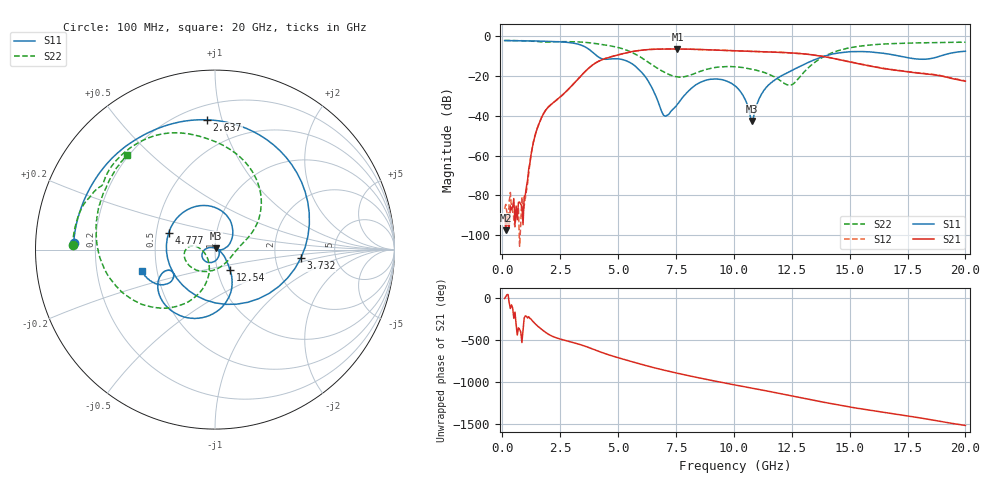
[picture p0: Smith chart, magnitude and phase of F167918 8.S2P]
!  2-Port S-parameters saved by WinCal
! VAR MeasName=S-Parameters (CALIBRATED_DATA) read from VNA (N5242A)
! VAR MeasDate=2016-11-22 10:25:13
! VAR NAME=F167918 8
! VAR FILENAME=F167918 8.S2P
! VAR DATE=2016-11-22 10:25:13
! VAR PHYS_PORTS=1,2
# Hz S DB R 50
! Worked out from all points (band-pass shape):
!   401 points, 100 MHz to 20 GHz, reference 50 ohm
!   highest |S21| = -6.30 dB at 7.562 GHz (marker M1); lowest = -97.6 dB at 149.8 MHz (marker M2)
!   |S21| within 3 dB of the highest: 4.991 GHz to 13.42 GHz (8.428 GHz wide, 91.6 % of centre)
!   lowest |S11| = -42.5 dB at 10.8 GHz (marker M3), VSWR 1.02, Z = 50.4 + j0.636 ohm
!   |S11| at or under -10 dB: 4.114 GHz to 13.89 GHz (9.773 GHz wide, 109 % of centre); 17.2 GHz to 18.88 GHz (1.672 GHz wide, 9.27 % of centre)
!   |S22| runs from -24.6 to -2.0 dB; largest |S21 - S12| = 0.0042
!   S11 on the Smith chart (normalised r, x): 100 MHz: 0.12, +0.02; 2.637 GHz: 0.29, +0.90; 3.732 GHz: 2.80, -0.35; 4.777 GHz: 0.58, +0.12; 12.54 GHz: 1.15, -0.27; 20 GHz: 0.41, -0.12
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1e8  -2.07 177.3  -90.07 -3.9  -86.70 139.0  -2.00 178.3
1.4975e8  -2.07 176.0  -97.64 17.1  -84.56 -45.2  -2.01 177.4
9.4575e8  -2.19 154.6  -80.71 122.4  -85.23 -175.1  -2.16 163.7
1.5925e9  -2.33 135.4  -43.68 11.1  -43.64 9.9  -2.59 153.3
2.63725e9  -2.80 93.5  -29.04 -139.4  -29.05 -140.0  -2.60 137.9
3.43325e9  -4.48 32.8  -19.38 159.5  -19.40 159.3  -2.83 119.5
3.73175e9  -6.37 -5.7  -15.94 130.7  -15.95 130.8  -3.12 111.5
4.12975e9  -10.14 -78.8  -12.66 88.7  -12.62 88.6  -3.74 100.6
4.7765e9  -11.23 160.3  -9.96 27.4  -9.93 27.0  -4.97 81.4
5.92075e9  -16.85 46.2  -7.03 -63.9  -7.05 -64.0  -10.05 37.5
6.7665e9  -34.13 -3.0  -6.36 -125.3  -6.37 -125.4  -16.50 10.4
7.065e9  -40.17 25.4  -6.30 -145.0  -6.32 -145.1  -18.37 -1.2
7.5625e9  -34.09 -8.0  -6.30 -176.5  -6.32 -176.5  -20.34 -33.9
8.7565e9  -22.14 -111.8  -6.63 113.2  -6.62 113.2  -16.78 -124.2
1.005e10  -24.86 179.9  -7.20 43.6  -7.22 43.6  -15.26 -171.9
1.079625e10  -42.54 57.7  -7.51 4.6  -7.50 4.8  -16.49 174.6
1.139325e10  -25.65 -31.6  -7.73 -26.5  -7.72 -26.4  -18.49 170.2
1.25375e10  -16.94 -54.1  -8.31 -87.8  -8.32 -87.7  -24.07 -133.6
1.338325e10  -12.18 -68.3  -9.22 -135.2  -9.19 -134.8  -14.05 -105.5
1.4826e10  -7.85 -109.3  -12.40 148.7  -12.26 149.1  -6.14 -140.5
1.67165e10  -8.93 -151.7  -16.53 66.7  -16.50 66.6  -3.67 178.4
2e10  -7.41 -163.5  -22.49 -79.7  -22.35 -80.4  -2.87 132.9
